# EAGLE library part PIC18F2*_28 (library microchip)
USB Microcontrollers with nanoWatt Technology High-Performance, Enhanced Flash, 28/40/44-Pin, Source: http://ww1.microchip.com/downloads/en/devicedoc/39632c.pdf
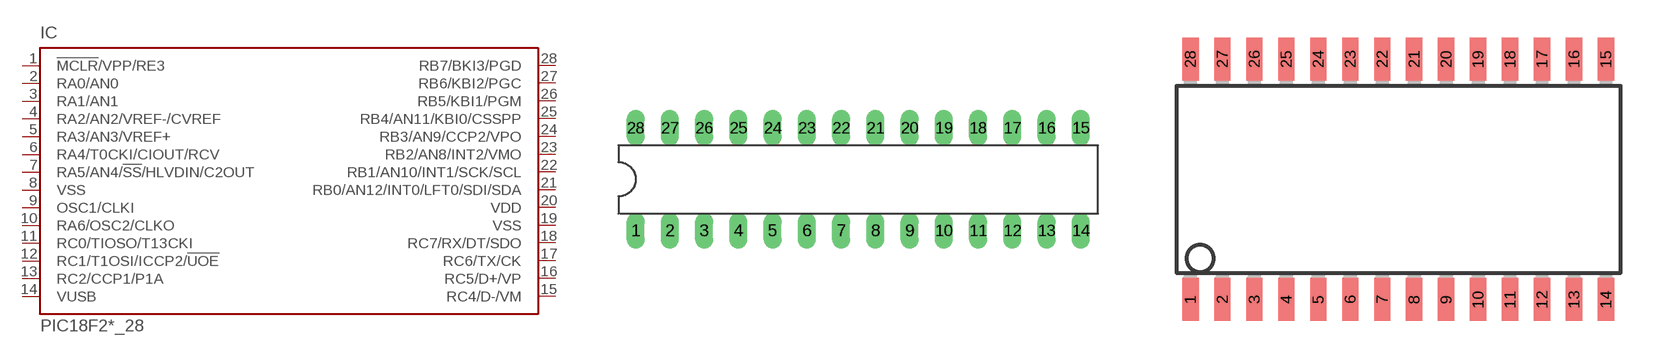
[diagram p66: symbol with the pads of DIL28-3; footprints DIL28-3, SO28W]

Designator prefix IC

## PIC18F2455_28DIP (MF: MICROCHIP; MPN: PIC18F2455-I/SP; OC_FARNELL: 1579600; OC_NEWARK: 01M8485), PIC18F2550_28DIP (MF: MICROCHIP; MPN: PIC18F2550-I/SP; OC_FARNELL: 1523822; OC_NEWARK: 80K6054)  [DIL28-3]
1  !MCLR!/VPP/RE3  in
2  RA0/AN0
3  RA1/AN1
4  RA2/AN2/VREF-/CVREF
5  RA3/AN3/VREF+
6  RA4/T0CKI/CIOUT/RCV
7  RA5/AN4/!SS!/HLVDIN/C2OUT
8  VSS  pwr
9  OSC1/CLKI  in
10  RA6/OSC2/CLKO  out
11  RC0/TIOSO/T13CKI
12  RC1/T1OSI/ICCP2/!UOE
13  RC2/CCP1/P1A
14  VUSB
15  RC4/D-/VM
16  RC5/D+/VP
17  RC6/TX/CK
18  RC7/RX/DT/SDO
19  VSS  pwr
20  VDD  pwr
21  RB0/AN12/INT0/LFT0/SDI/SDA
22  RB1/AN10/INT1/SCK/SCL
23  RB2/AN8/INT2/VMO
24  RB3/AN9/CCP2/VPO
25  RB4/AN11/KBI0/CSSPP
26  RB5/KBI1/PGM
27  RB6/KBI2/PGC
28  RB7/BKI3/PGD

## PIC18F2455_28W (MF: MICROCHIP; MPN: PIC18F2455-I/SO; OC_FARNELL: 1579598; OC_NEWARK: 64J3768), PIC18F2550_28W (MF: MICROCHIP; MPN: PIC18F2550-I/SO; OC_FARNELL: 9321268; OC_NEWARK: 73K1297)  [SO28W]
Pads as for DIL28-3

## Footprint DIL28-3 (pad centres in mm)
Dual In Line package type P
drill 0.813 long: 1 -16.51,-3.81; 2 -13.97,-3.81; 3 -11.43,-3.81; 4 -8.89,-3.81; 5 -6.35,-3.81; 6 -3.81,-3.81; 7 -1.27,-3.81; 8 1.27,-3.81; 9 3.81,-3.81; 10 6.35,-3.81; 11 8.89,-3.81; 12 11.43,-3.81; 13 13.97,-3.81; 14 16.51,-3.81; 15 16.51,3.81; 16 13.97,3.81; 17 11.43,3.81; 18 8.89,3.81; 19 6.35,3.81; 20 3.81,3.81; 21 1.27,3.81; 22 -1.27,3.81; 23 -3.81,3.81; 24 -6.35,3.81; 25 -8.89,3.81; 26 -11.43,3.81; 27 -13.97,3.81; 28 -16.51,3.81

## Footprint SO28W (pad centres in mm)
28-Lead Plastic Small Outline (SO) Wide, 300 mil Body (SOIC) Source: http://ww1.microchip.com/downloads/en/devicedoc/39632c.pdf
smd 0.65 x 1.7: 1 -7.62,-4.78; 2 -6.35,-4.78; 3 -5.08,-4.78; 4 -3.81,-4.78; 5 -2.54,-4.78; 6 -1.27,-4.78; 7 0,-4.78; 8 1.27,-4.78; 9 2.54,-4.78; 10 3.81,-4.78; 11 5.08,-4.78; 12 6.35,-4.78; 13 7.62,-4.78; 14 8.89,-4.78; 15 8.89,4.78; 16 7.62,4.78; 17 6.35,4.78; 18 5.08,4.78; 19 3.81,4.78; 20 2.54,4.78; 21 1.27,4.78; 22 0,4.78; 23 -1.27,4.78; 24 -2.54,4.78; 25 -3.81,4.78; 26 -5.08,4.78; 27 -6.35,4.78; 28 -7.62,4.78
